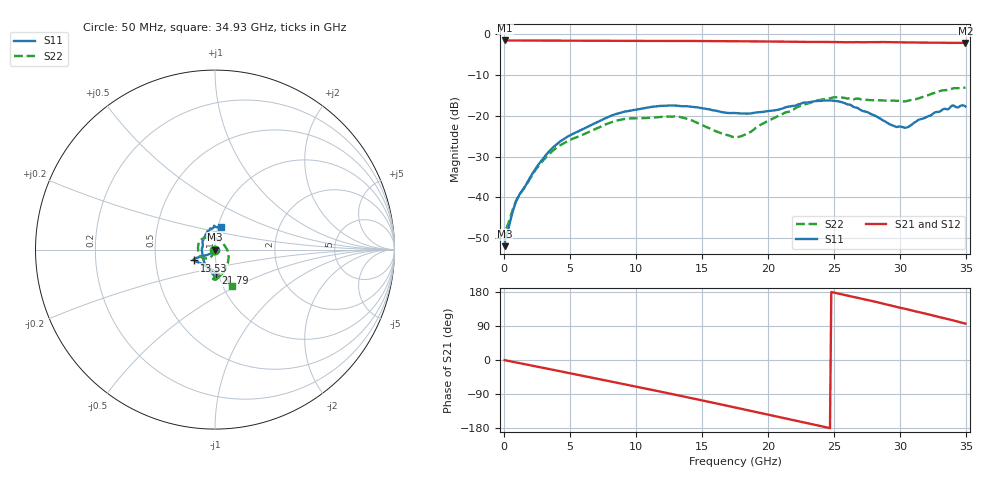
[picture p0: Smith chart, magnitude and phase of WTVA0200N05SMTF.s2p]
! 50 ohm 2-Port S-parameters measured by Modelithics Inc support@modelithics.com  Tampa, FL USA 813-866-6335 (February 2024)
! Smiths Interconnect,  2dB P/N: WTVA0200N05SMTF, Temperature: 50 C
! Board: 10 mil Rogers 4350B, Mounting Pad Dimensions: Length: 15 mils, Width: 25 mils, Gap: 40 mils.
# Hz S RI R 50
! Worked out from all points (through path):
!   352 points, 50 MHz to 34.93 GHz, reference 50 ohm
!   highest |S21| = -1.65 dB at 100 MHz (marker M1); lowest = -2.3 dB at 34.93 GHz (marker M2)
!   group delay of S21, straight-line fit = 20.8 ps
!   lowest |S11| = -51.9 dB at 50 MHz (marker M3), VSWR 1.01, Z = 49.7 + j0.0278 ohm
!   |S11| at or under -10 dB: start of sweep to end of sweep
!   |S22| runs from -50.6 to -13.1 dB; largest |S21 - S12| = 0.0095
!   S11 on the Smith chart (normalised r, x): 50 MHz: 0.99, +0.00; 13.53 GHz: 0.79, -0.10; 21.79 GHz: 0.97, -0.26; 34.93 GHz: 1.04, +0.26
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5e7  -0.00253 0.00028  0.8266 -0.00448  0.8259 -0.0045  -0.0029 -0.000565
1e8  -0.00301 -0.000806  0.8268 -0.0102  0.8262 -0.0103  -0.00362 -0.00117
8.965e8  -0.0058 -0.00661  0.821 -0.0905  0.8204 -0.091  -0.00502 -0.00742
2.389e9  -0.0157 -0.016  0.7894 -0.2366  0.7888 -0.2363  -0.0079 -0.02
3.782e9  -0.0329 -0.0258  0.7384 -0.366  0.7377 -0.3662  -0.0167 -0.0344
5.8715e9  -0.0581 -0.0337  0.6198 -0.541  0.6196 -0.5405  -0.0336 -0.0466
8.8565e9  -0.0993 -0.0443  0.382 -0.7233  0.3805 -0.7234  -0.0803 -0.0393
1.1742e10  -0.119 -0.0543  0.1029 -0.8085  0.1017 -0.8081  -0.0947 0.0163
1.3533e10  -0.1149 -0.0606  -0.0813 -0.8111  -0.0826 -0.8105  -0.0755 0.0568
1.54235e10  -0.0974 -0.0702  -0.2752 -0.7658  -0.2776 -0.7642  -0.0214 0.0682
1.7513e10  -0.0634 -0.0867  -0.4697 -0.6605  -0.4695 -0.6601  0.0362 0.0406
1.8508e10  -0.0432 -0.0964  -0.5495 -0.59  -0.5495 -0.5896  0.0595 0.0128
1.96025e10  -0.0227 -0.1082  -0.6269 -0.5038  -0.6266 -0.5034  0.0748 -0.0276
2.17915e10  0.00416 -0.1308  -0.7376 -0.3016  -0.7372 -0.3006  0.0629 -0.0993
2.33835e10  0.0135 -0.1478  -0.7811 -0.1413  -0.7803 -0.1414  0.0329 -0.143
2.55725e10  -0.00518 -0.1456  -0.7827 0.0944  -0.7816 0.0965  -0.00681 -0.1661
2.7861e10  -0.0475 -0.0915  -0.7181 0.3254  -0.7156 0.3281  -0.00779 -0.1538
2.91545e10  -0.0682 -0.0393  -0.6451 0.4536  -0.6403 0.4588  0.00754 -0.1511
3.0448e10  -0.0687 0.0186  -0.5469 0.5579  -0.5415 0.562  0.0308 -0.147
3.1443e10  -0.0634 0.0634  -0.4591 0.6278  -0.4558 0.6289  0.0523 -0.1553
3.39305e10  -0.00431 0.1327  -0.2036 0.7451  -0.1983 0.7456  0.0855 -0.1953
3.49255e10  0.035 0.1242  -0.0831 0.7649  -0.083 0.7638  0.0922 -0.2002
